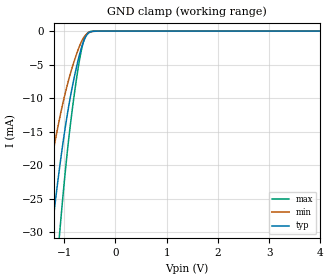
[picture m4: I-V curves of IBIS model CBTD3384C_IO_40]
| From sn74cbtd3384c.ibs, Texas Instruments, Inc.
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[Model]   CBTD3384C_IO_40
Model_type  Terminator
| variable   typ   min   max
C_comp   7.09pF   4.34pF   14.74pF
| C_tri-state   7.09pF   4.34pF   14.74pF
[Temperature Range]   40   100   -40
| Ambient temperature   25   85   -40
[Voltage range]   4   4   4
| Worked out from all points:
|   GND clamp passes 1 mA (typ) near -0.59 V on its own axis
[GND Clamp]
| CBTD3384C_IO_40
|   Voltage   I(typ)   I(min)   I(max)
-5V       -402.2mA   -300.9mA   -511.8mA
-1.48V    -47.52mA   -30.69mA   -70.1mA
-1.455V   -45.58mA   -29.39mA   -67.35mA
-1.23V    -29.29mA   -18.74mA   -43.72mA
-1.085V   -20.21mA   -12.94mA   -30.02mA
-930mV    -12.11mA   -7.817mA   -17.51mA
-845mV    -8.525mA   -5.511mA   -11.99mA
-760mV    -5.441mA   -3.499mA   -7.23mA
-695mV    -3.394mA   -2.169mA   -4.131mA
-630mV    -1.756mA   -1.13mA    -1.802mA
-515mV    -258.9uA   -204.1uA   -139.2uA
4V        419.1pA    1.535nA    94.95pA
